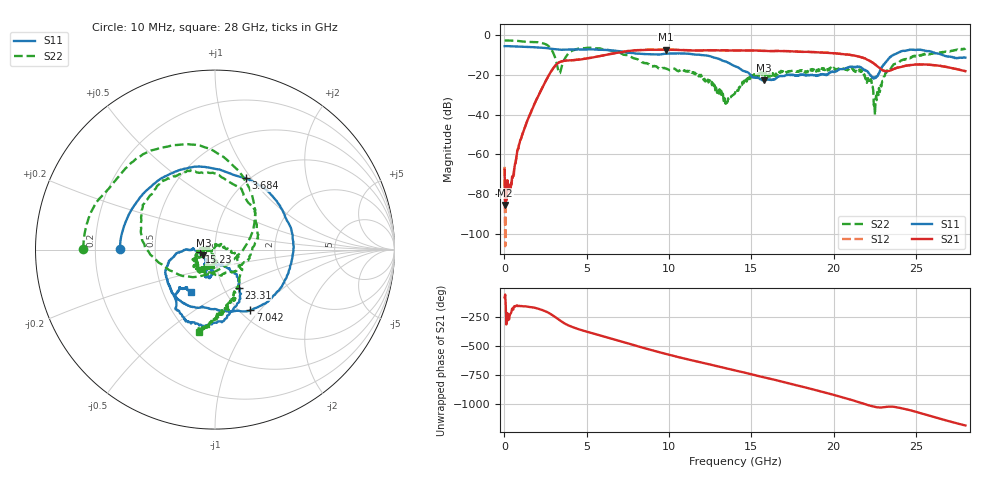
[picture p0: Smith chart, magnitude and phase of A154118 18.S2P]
!  2-Port S-parameters saved by WinCal
! VAR MeasName=S-Parameters (CALIBRATED_DATA) read from VNA (N5230A)
! VAR MeasDate=2015-9-10 14:35:47
! VAR NAME=A154118 18
! VAR FILENAME=A154118 18.S2P
! VAR DATE=2015-9-10 14:35:47
! VAR PHYS_PORTS=1,2
# Hz S DB R 50
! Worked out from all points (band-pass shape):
!   801 points, 10 MHz to 28 GHz, reference 50 ohm
!   highest |S21| = -7.29 dB at 9.806 GHz (marker M1); lowest = -85.5 dB at 44.99 MHz (marker M2)
!   |S21| within 3 dB of the highest: 5.97 GHz to 21.27 GHz (15.3 GHz wide, 112 % of centre)
!   lowest |S11| = -22.8 dB at 15.75 GHz (marker M3), VSWR 1.16, Z = 43.8 - j2.82 ohm
!   |S11| at or under -10 dB: 11.95 GHz to 23.61 GHz (11.66 GHz wide, 65.6 % of centre); 26.62 GHz to end of sweep
!   |S22| runs from -40.3 to -2.7 dB; largest |S21 - S12| = 0.0079
!   S11 on the Smith chart (normalised r, x): 10 MHz: 0.31, +0.00; 3.684 GHz: 0.96, +0.94; 7.042 GHz: 1.11, -0.89; 15.23 GHz: 0.84, -0.02; 23.31 GHz: 1.18, -0.53; 28 GHz: 0.69, -0.35
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1e7  -5.55 179.6  -67.83 -81.0  -66.30 9.4  -2.68 179.8
4.49875e7  -5.54 178.6  -85.54 -56.9  -106.24 -67.5  -2.69 178.9
4.2985e8  -5.61 166.6  -75.05 157.2  -75.34 178.9  -2.75 169.5
1.024638e9  -5.84 149.4  -51.65 -156.4  -51.62 -156.9  -3.12 154.9
2.424138e9  -6.43 106.3  -24.41 162.4  -24.40 162.5  -4.30 105.2
3.053912e9  -7.07 85.4  -15.67 111.3  -15.67 111.4  -10.72 39.9
3.333812e9  -7.32 77.7  -13.66 82.0  -13.63 82.0  -19.19 -51.7
3.683688e9  -7.28 66.8  -12.87 50.9  -12.87 51.1  -11.66 -151.5
4.698325e9  -7.26 28.3  -12.15 -4.9  -12.13 -4.8  -6.51 145.6
7.042488e9  -8.15 -59.9  -8.69 -99.9  -8.61 -100.0  -8.99 64.3
9.351662e9  -9.77 -102.5  -7.38 166.9  -7.31 166.6  -16.71 -57.7
9.8065e9  -9.37 -108.5  -7.29 149.8  -7.26 149.4  -16.79 -85.2
1.34452e10  -13.28 -174.7  -7.69 26.1  -7.64 25.5  -34.55 -173.4
1.4005e10  -15.63 179.9  -7.73 7.4  -7.70 6.9  -29.21 -104.4
1.522956e10  -21.38 -171.6  -7.74 -34.4  -7.73 -35.0  -20.87 -97.5
1.575438e10  -22.83 -153.7  -7.94 -52.4  -7.92 -52.8  -20.13 -113.5
1.869332e10  -19.92 -114.5  -8.52 -155.1  -8.53 -155.4  -17.08 -115.3
2.163228e10  -16.16 -109.7  -11.06 87.9  -11.02 86.9  -18.52 -154.5
2.257694e10  -21.31 -74.9  -15.19 49.8  -15.10 49.2  -30.49 90.0
2.331168e10  -12.06 -58.0  -18.08 53.8  -17.99 52.7  -17.67 -17.4
2.334666e10  -11.72 -57.2  -18.01 54.2  -17.93 53.3  -17.25 -17.1
2.8e10  -11.29 -119.8  -18.12 -108.5  -18.20 -109.4  -6.64 -101.1
